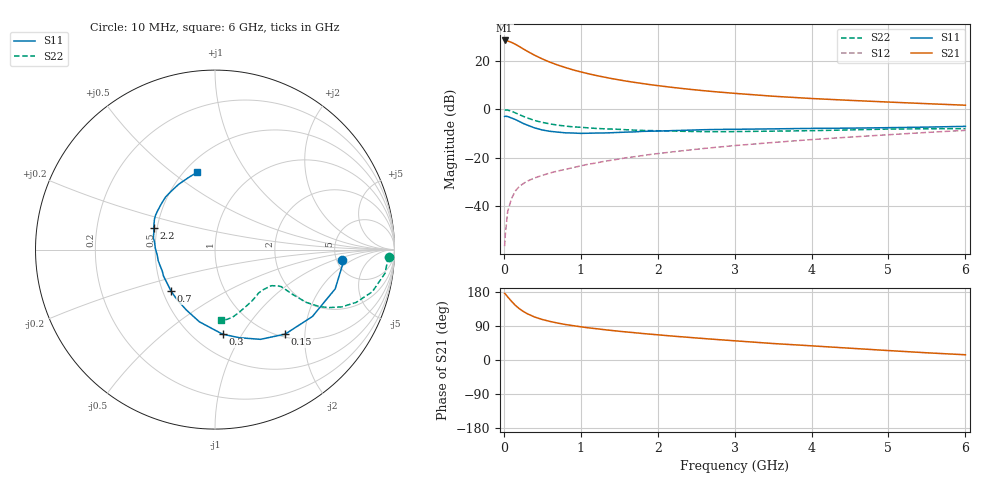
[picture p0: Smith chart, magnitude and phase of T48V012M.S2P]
! Infineon Technologies  Discrete & RF Semiconductors
! BFR182T
! Si NPN RF Bipolar Junction Transistor in SC75
! VCE = 8 V  IC = 12 mA
! Common Emitter S-Parameters:  October  1999
# GHz  S  MA  R  50
!  f  S11  S21  S12  S22
! GHz  MAG  ANG  MAG  ANG  MAG  ANG  MAG  ANG
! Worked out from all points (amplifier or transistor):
!   36 points, 10 MHz to 6 GHz, reference 50 ohm
!   highest |S21| = 28.3 dB at 10 MHz (marker M1)
!   |S21| within 3 dB of that: start of sweep to 227.3 MHz
!   unconditionally stable (mu >= 1): 998.1 MHz to 3.937 GHz
!   at 250 MHz: K = 0.47, MSG = 27.8 dB, |S12| = -30.7 dB
!   at 1.4 GHz: K = 1.06, MAG = 15.3 dB, |S12| = -21.0 dB
!   at 6 GHz: K = 0.87, MSG = 5.2 dB, |S12| = -8.7 dB
!   S11 on the Smith chart (normalised r, x): 10 MHz: 5.55, -1.23; 150 MHz: 1.06, -1.59; 300 MHz: 0.68, -0.83; 700 MHz: 0.55, -0.29; 2.2 GHz: 0.48, +0.13; 6 GHz: 0.58, +0.62
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0.01  0.7072 -4.5  26.12 175.7  0.0015 70.3  0.9675 -2.3
0.02  0.7176 -5.9  26.07 174.3  0.0027 95.4  0.965 -3.2
0.05  0.7045 -18.1  25.5 166.5  0.0078 83.3  0.9565 -7.9
0.1  0.6583 -34.5  23.83 154.9  0.0144 75.1  0.9074 -15.0
0.15  0.612 -50.3  21.79 144.2  0.0206 69.2  0.8396 -20.5
0.2  0.5606 -63.1  19.64 135.6  0.0255 66.0  0.7753 -24.3
0.25  0.5099 -74.4  17.59 128.6  0.0291 62.8  0.7138 -26.9
0.3  0.4731 -84.9  15.79 122.6  0.0326 61.2  0.6647 -28.6
0.4  0.4116 -102.2  12.95 113.4  0.0383 60.1  0.5847 -30.1
0.5  0.3724 -115.4  10.87 106.9  0.0432 60.2  0.5342 -30.0
0.6  0.3498 -127.2  9.306 101.7  0.0484 61.0  0.4968 -30.0
0.7  0.3368 -136.7  8.14 97.4  0.0532 62.4  0.4693 -29.7
0.9  0.3226 -152.8  6.466 90.6  0.0625 63.9  0.4325 -29.4
1.1  0.3195 -164.9  5.376 84.8  0.0735 64.7  0.4117 -29.7
1.3  0.3233 -174.4  4.602 80.2  0.0839 65.4  0.3946 -30.6
1.6  0.3372 174.6  3.773 73.8  0.1001 66.2  0.3761 -32.3
2.2  0.3618 160.5  2.802 63.0  0.1323 66.3  0.3541 -38.1
2.8  0.3825 150.2  2.251 53.6  0.166 64.9  0.3428 -45.3
3.5  0.3928 139.7  1.85 43.5  0.206 62.6  0.3527 -54.4
4.5  0.4067 126.8  1.52 31.1  0.2661 58.1  0.3739 -68.7
5.5  0.4273 110.5  1.299 19.0  0.3318 52.7  0.3948 -80.7
6  0.4429 102.8  1.208 13.8  0.3658 49.4  0.396 -85.5
